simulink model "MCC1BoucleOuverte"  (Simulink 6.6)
settings: Solver=ode45  StartTime=0.0  StopTime=0.4  RelTol=1e-3
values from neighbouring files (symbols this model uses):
  Cr = Cmax/4    (= 0.0068445)    [moteur.m]
  h = 50e-6    (= 5e-05)    [moteur.m]
  J = 2e-6    (= 2e-06)    [moteur.m]
  K = 0.0234    [moteur.m]
  kv = 13e-6    (= 1.3e-05)    [moteur.m]
  L = 0.000238    [moteur.m]
  omegaref = 300    [moteur.m]
  R = 2.19    [moteur.m]
libraries: simulink x1

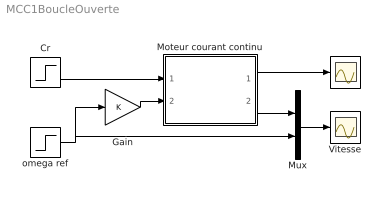
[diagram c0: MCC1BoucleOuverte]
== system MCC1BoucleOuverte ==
  Cr : Step  Time=0.25  After=Cr  SampleTime=0
  Gain : Gain  Gain=K
  I : Scope
  Moteur courant continu : Subsystem
  Mux : Mux  Inputs=2
  Vitesse : Scope
  omega ref : Step  Time=0.05  After=omegaref  SampleTime=0
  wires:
  omega ref/1 -> Gain/1, Mux/2
  Gain/1 -> Moteur courant continu/2(Uref)
  Mux/1 -> Vitesse/1
  Cr/1 -> Moteur courant continu/1(Cr)
  Moteur courant continu/1(I) -> I/1
  Moteur courant continu/2(omega) -> Mux/1

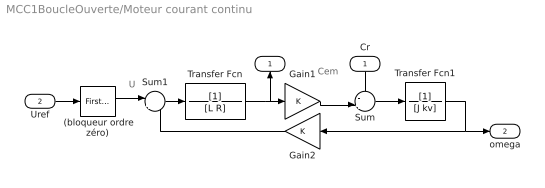
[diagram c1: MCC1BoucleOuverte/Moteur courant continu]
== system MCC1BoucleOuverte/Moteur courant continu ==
  note: U
  note: I
  note: Cem
  Cr : Inport  Orientation=down
  Uref : Inport  Port=2
  " (bloqueur ordre zéro)" : simulink/Discrete/First-Order Hold  SystemSampleTime=-1  Ts=h
  Gain1 : Gain  Gain=K
  Gain2 : Gain  Orientation=left  Gain=K
  Sum : Sum  Inputs=-+|
  Sum1 : Sum  Inputs=|+-
  Transfer Fcn : TransferFcn  Denominator=[L R]
  Transfer Fcn1 : TransferFcn  Denominator=[J kv]
  I : Outport  Orientation=up
  omega : Outport  Port=2
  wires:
  Transfer Fcn/1 -> Gain1/1, I/1
  Gain1/1 -> Sum/2
  Sum/1 -> Transfer Fcn1/1
  Transfer Fcn1/1 -> Gain2/1, omega/1
  " (bloqueur ordre zéro)"/1 -> Sum1/1
  Sum1/1 -> Transfer Fcn/1
  Gain2/1 -> Sum1/2
  Cr/1 -> Sum/1
  Uref/1 -> " (bloqueur ordre zéro)"/1
